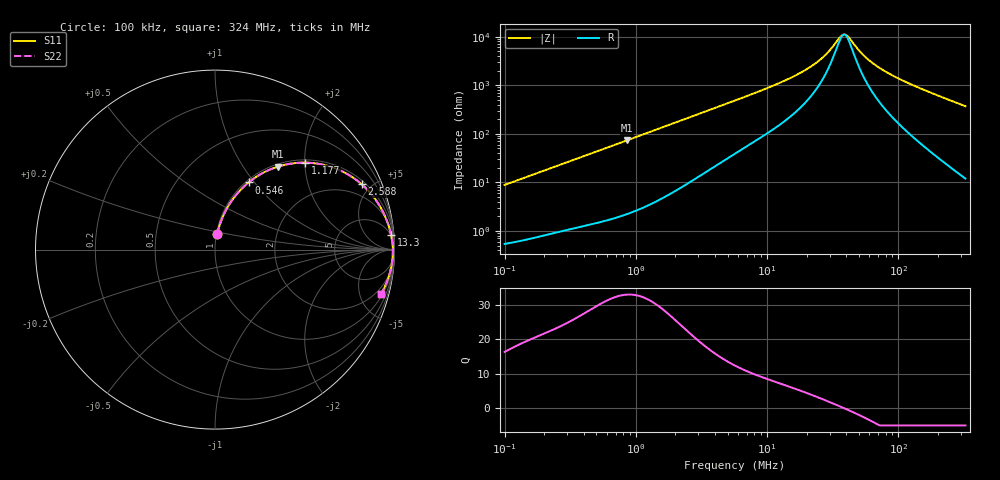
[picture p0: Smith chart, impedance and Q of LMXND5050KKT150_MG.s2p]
! LMXND5050KKT150_MG  S-PARAMETER MODEL  ( General Type )
! Model Generated by TAIYO YUDEN Corporation (http://www.ty-top.com)
! Version 1.0
! TAIYO YUDEN Control No. 191023NI43SB-FBB
! Copyright(c) 2019 TAIYO YUDEN CO.,LTD. All Rights Reserved.
! Product Description (link to TY-COMPAS)
! https://ds.yuden.co.jp/TYCOMPAS/or/detail?pn=LMXND5050KKT150MMG&u=M
! Products Name : Inductors
! Characteristics :
!  Inductance : 15 uH , SRF(min) : 19 MHz , DC Resistance(max) : 0.48 Ohm
!  Rated Current : Saturation :680 mA , Temp Rise : 650 mA
!  Case Size : 4.9 x 4.9 / 0.193 x 0.193 [mm/inch] , Thickness : 1 / 0.039 [mm/inch]
!  (Conditions: Temperature = 25 degC , DC Bias Current/Voltage = 0A / 0V)
! External Node Assignments :
!  1  o---GGG---o  2
! GND o---------o GND
! Frequency Range : 0.1MHz  -  324.04089MHz  [ 402 STEP ]
# MHz S RI R 50
! Freq[MHz].  S11 Real  S11 Imag  S21 Real  S21 Imag  S12 Real  S12 Imag  S22 Real  S22 Imag
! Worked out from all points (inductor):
!   401 points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, 100 kHz to 324 MHz, reference 50 ohm
!   read as one part in series: L = 14 uH near 104.1 kHz
!   highest Q = 33 at 851.7 kHz (marker M1), where L = 13.6 uH
!   self-resonance near 38.04 MHz
!   S11 on the Smith chart (normalised r, x): 100 kHz: 1.01, +0.18; 546 kHz: 1.03, +0.93; 1.177 MHz: 1.06, +2.00; 2.588 MHz: 1.20, +4.39; 13.3 MHz: 4, +24; 324 MHz: 1.24, -7.37
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0.1  0.0129 0.0865  0.9871 -0.0865  0.9871 -0.0865  0.0129 0.0865
0.198793  0.0364 0.1656  0.9636 -0.1656  0.9636 -0.1656  0.0364 0.1656
0.38728  0.1087 0.2934  0.8913 -0.2934  0.8913 -0.2934  0.1087 0.2934
0.546042  0.1874 0.3741  0.8126 -0.3741  0.8126 -0.3741  0.1874 0.3741
0.851744  0.3499 0.462  0.6501 -0.462  0.6501 -0.462  0.3499 0.462
1.176882  0.5011 0.4846  0.4989 -0.4846  0.4989 -0.4846  0.5011 0.4846
1.499861  0.6157 0.4698  0.3843 -0.4698  0.3843 -0.4698  0.6157 0.4698
2.588311  0.8174 0.364  0.1826 -0.364  0.1826 -0.364  0.8174 0.364
3.723861  0.8952 0.2778  0.1048 -0.2778  0.1048 -0.2778  0.8952 0.2778
5.692459  0.9446 0.1918  0.0554 -0.1918  0.0554 -0.1918  0.9446 0.1918
13.30188  0.9817 0.0796  0.0183 -0.0796  0.0183 -0.0796  0.9817 0.0796
22.04577  0.9886 0.0376  0.0114 -0.0376  0.0114 -0.0376  0.9886 0.0376
27.53385  0.9901 0.0221  0.00994 -0.0221  0.00994 -0.0221  0.9901 0.0221
35.80646  0.9909 0.00491  0.00907 -0.00491  0.00907 -0.00491  0.9909 0.00491
38.82106  0.991 -0.000276  0.00895 0.000276  0.00895 0.000276  0.991 -0.000276
42.08946  0.9911 -0.00547  0.0089 0.00547  0.0089 0.00547  0.9911 -0.00547
50.48494  0.991 -0.0174  0.00904 0.0174  0.00904 0.0174  0.991 -0.0174
58.15638  0.9906 -0.027  0.00939 0.027  0.00939 0.027  0.9906 -0.027
69.75669  0.9898 -0.0402  0.0102 0.0402  0.0102 0.0402  0.9898 -0.0402
85.37896  0.9883 -0.0564  0.0117 0.0564  0.0117 0.0564  0.9883 -0.0564
150.3463  0.9779 -0.1154  0.0221 0.1154  0.0221 0.1154  0.9779 -0.1154
324.0409  0.9246 -0.2483  0.0754 0.2483  0.0754 0.2483  0.9246 -0.2483
